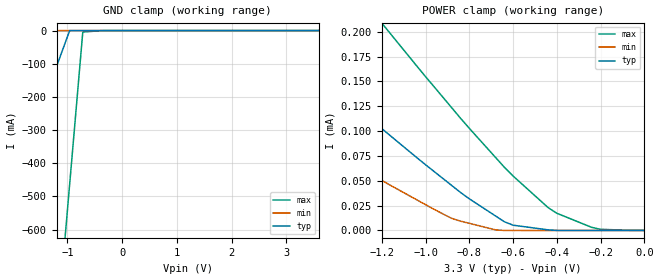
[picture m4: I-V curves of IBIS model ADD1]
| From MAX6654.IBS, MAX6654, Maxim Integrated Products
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|   ADD1 Input
[Model]   ADD1
|Signals   ADD1
Model_type   Input
Vinl = 0.8V
Vinh = 2.2V
C_comp   2.150E-12   1.833E-12   2.461E-12
[Temperature Range]   25   -55   125
[Voltage Range]   3.30V   3.00V   3.60V
[Pullup Reference]   3.30V   3.00V   3.60V
[Pulldown Reference]   0.00V   0.00V   0.00V
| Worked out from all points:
|   GND clamp passes 1 mA (typ) near -0.96 V on its own axis
[POWER_clamp]
| Note that the [POWER_clamp] voltage table is referenced to Vcc
| and is calculated using Vtable=Vcc - Vmeasured.
|V(V)   I(typ)   I(min)   I(max)
-3.6V     557.5uA    358.6uA    884uA
-2.4V     328.3uA    203.5uA    543.4uA
-2.36V    320.7uA    198.3uA    532.1uA
-1.76V    207uA      121.2uA    363.5uA
-1.72V    199.5uA    116.1uA    352.3uA
-1.2V     102.5uA    50.35uA    208.7uA
-1.16V    95.18uA    45.38uA    197.9uA
-880mV    45.2uA     12.12uA    123.4uA
-640mV    8.788uA    24.23nA    63.67uA
-440mV    616.6nA    167pA      23.04uA
-240mV    3.047nA    150.7pA    3.099uA
0V        76.8pA     60.27pA    84.95nA
[GND_clamp]
| Note that the [GND_clamp] voltage table is referenced to Gnd.
|V(V)   I(typ)   I(min)   I(max)
-3.6V     -1.191A    -1.422mA   -5.514A
-2.32V    -613.6mA   -732.7uA   -3.065A
-2.24V    -577.5mA   -689.6uA   -2.912A
-1.04V    -36.16mA   -43.14uA   -616.5mA
-960mV    -112.7uA   -47.8nA    -463.5mA
-720mV    -45.14uA   -18.91nA   -4.368mA
-320mV    -30.04nA   240.5pA    -13.96uA
3.6V      706.8pA    1.03nA     85.07nA
